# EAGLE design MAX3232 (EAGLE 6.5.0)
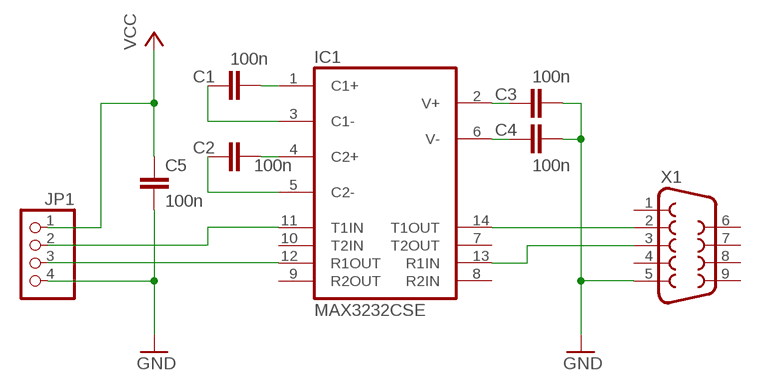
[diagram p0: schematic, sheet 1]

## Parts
C1  100n  C-EUC1206  [C1206]
C2  100n  C-EUC1206  [C1206]
C3  100n  C-EUC1206  [C1206]
C4  100n  C-EUC1206  [C1206]
C5  100n  C-EUC1206  [C1206]
IC1  MAX3232CSE  [SO16]
JP1  PINHD-1X4  [1X04]
X1  F09HP  [F09HP]

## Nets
GND: C3.2 C4.2 C5.2 JP1.4 X1.5
N$1: C1.2 IC1.1(C1+)
N$2: C1.1 IC1.3(C1-)
N$3: C2.2 IC1.4(C2+)
N$4: C2.1 IC1.5(C2-)
N$5: C3.1 IC1.2(V+)
N$6: C4.1 IC1.6(V-)
N$8: IC1.14(T1OUT) X1.2
N$9: IC1.13(R1IN) X1.3
N$10: IC1.11(T1IN) JP1.2
N$11: IC1.12(R1OUT) JP1.3
VCC: C5.1 JP1.1
Unconnected: IC1.7(T2OUT) IC1.8(R2IN) IC1.9(R2OUT) IC1.10(T2IN) X1.1 X1.4 X1.6 X1.7 X1.8 X1.9

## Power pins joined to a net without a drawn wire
GND: IC1.15(GND)
VCC: IC1.16(VCC)

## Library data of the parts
C1-C5 = rcl:C-EU: CAPACITOR, European symbol
IC1 = maxim:MAX3232*: True RS-232 Transceivers 3.0V to 5.5V, Low-Power up to 1Mbps, Using Four 0.1µF External Capacitors Source: http://pdfserv.maxim-ic.com/en/ds/MAX3222-MAX3241.pdf; MPN: MAX3232CSE; OC_FARNELL: 9725490; OC_NEWARK: 90C2890
JP1 = pinhead:PINHD-1X4: PIN HEADER
X1 = con-subd:F09: SUB-D; OC_FARNELL: unknown; OC_NEWARK: unknown

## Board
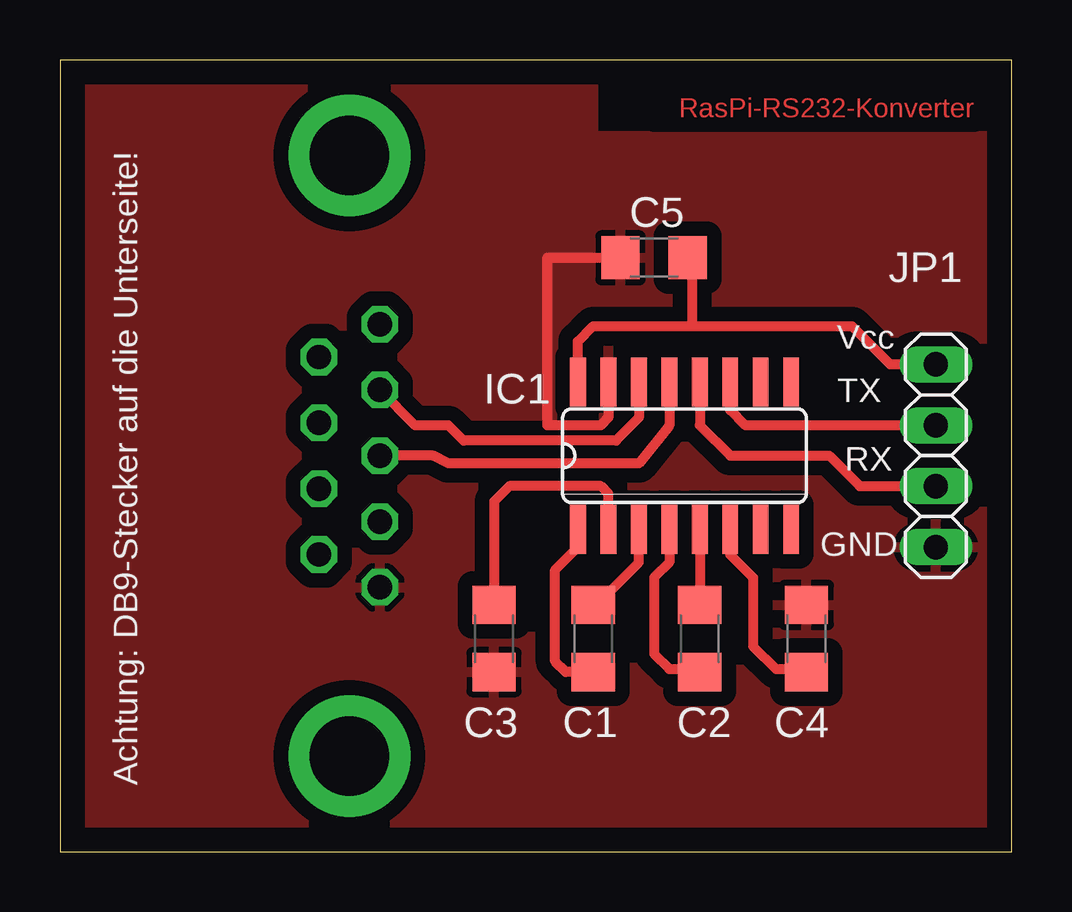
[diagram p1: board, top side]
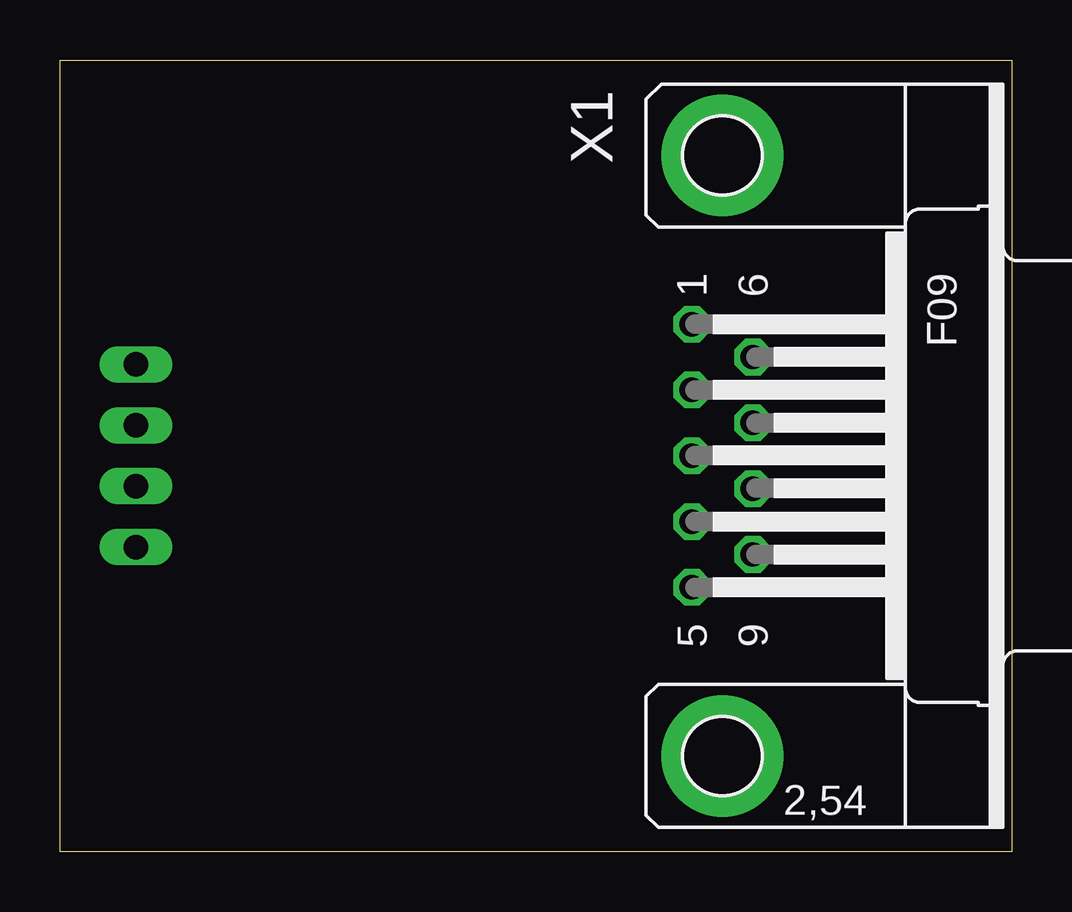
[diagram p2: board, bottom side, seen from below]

Size 39.67 x 33.01 mm. Coordinates in mm from the lower left corner, seen from the top.
Outline: 0,0 39.67,0 39.67,33.01 0,33.01 0,0
Copper layers (1*16): Top 0.035mm / dielectric 1.5mm / Bottom 0.035mm
Design rules "default": minimum track width 10mil, minimum drill 24mil, track to track 8mil, track to pad 8mil, pad to pad 8mil, via to via 8mil, smd to smd 8mil, copper to edge 40mil, drill to drill 8mil, minimum pad ring 10mil, minimum via ring 8mil, stop-mask expansion 4mil, vias tented up to drill 0mil, thermal gap 10mil

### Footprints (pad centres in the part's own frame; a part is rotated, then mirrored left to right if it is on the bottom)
C1206 = smd 1.6 x 1.8: 1 -1.4,0; 2 1.4,0
SO16 = smd 0.66 x 2.032: 1 -4.445,-3.073; 2 -3.175,-3.073; 3 -1.905,-3.073; 4 -0.635,-3.073; 5 0.635,-3.073; 6 1.905,-3.073; 7 3.175,-3.073; 8 4.445,-3.073; 9 4.445,3.073; 10 3.175,3.073; 11 1.905,3.073; 12 0.635,3.073; 13 -0.635,3.073; 14 -1.905,3.073; 15 -3.175,3.073; 16 -4.445,3.073
1X04 = drill 1.016 long: 1 -3.81,0; 2 -1.27,0; 3 1.27,0; 4 3.81,0
F09HP = drill 1.016 octagon: 1 -5.486,-1.27; 2 -2.743,-1.27; 3 0,-1.27; 4 2.743,-1.27; 5 5.486,-1.27; 6 -4.115,1.27; 7 -1.372,1.27; 8 1.372,1.27; 9 4.115,1.27 | drill 3.302 pad 5.08: G1 -12.522,0; G2 12.522,0

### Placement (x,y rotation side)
C1  22.23,8.89 270 top
C2  26.67,8.89 270 top
C3  18.1,8.89 270 top
C4  31.11,8.89 90 top
C5  24.77,24.77 180 top
IC1  26.04,16.51 0 top
JP1  36.51,16.51 270 top
X1  12.06,16.51 270 bottom

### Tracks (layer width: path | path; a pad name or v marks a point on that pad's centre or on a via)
GND
  Top 0.406: IC1.15 22.86,18.1 22.54,17.78 20.32,17.78 20.32,24.77 C5.2
  pour Top (isolate 0.61): 0.64,32.07 22.23,32.07 22.23,29.84 39.05,29.84 39.05,0.95 0.64,0.95
N$1
  Top 0.406: C1.2 21.09,7.49 20.64,7.94 20.64,11.75 21.59,12.7 IC1.1
N$2
  Top 0.406: C1.1 22.36,10.29 24.13,12.06 IC1.3
N$3
  Top 0.406: IC1.4 25.4,12.06 24.77,11.43 24.77,8.26 25.4,7.62 26.54,7.62 C2.2
N$4
  Top 0.406: IC1.5 C2.1
N$5
  Top 0.406: IC1.2 22.86,14.92 22.54,15.24 18.73,15.24 18.1,14.61 C3.1
N$6
  Top 0.406: IC1.6 27.94,12.38 28.89,11.43 28.89,8.57 29.84,7.62 30.98,7.62 C4.1
N$8
  Top 0.406: IC1.14 24.13,18.1 23.18,17.14 16.83,17.14 16.19,17.78 14.81,17.78 X1.2
N$9
  Top 0.406: IC1.13 25.4,17.78 24.13,16.19 16.19,16.19 15.56,16.51 X1.3
N$10
  Top 0.406: JP1.2 28.57,17.78 27.94,18.41 IC1.11
N$11
  Top 0.406: IC1.12 26.67,17.78 27.94,16.51 32.07,16.51 33.34,15.24 JP1.3
VCC
  Top 0.406: JP1.1 34.61,20.32 33.02,21.91 26.35,21.91 | IC1.16 21.59,21.27 22.23,21.91 26.35,21.91 | C5.1 26.35,24.13 26.35,21.91

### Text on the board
Top: RasPi-RS232-Konverter
tPlace: Achtung: DB9-Stecker auf die Unterseite! | Vcc | TX | RX | GND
